PROGRAM FastTask
VAR
	_iBuffer: UDINT := 0;
END_VAR

FOR _iBuffer := 0 TO MAX_CSV_RING_BUFFER BY 1 DO
	IF gCSV_Buffer[_iBuffer].bFull THEN
		gCSV_Buffer[_iBuffer].fbWriter(bWrite:= gCSV_Buffer[_iBuffer].bFull,sFileName:=gCSV_Buffer[_iBuffer].sPath, pBuffer :=ADR(gCSV_Buffer[_iBuffer].aBuffer));
		gCSV_Buffer[_iBuffer].bFull := gCSV_Buffer[_iBuffer].fbWriter.bBusy;
	END_IF
END_FOR

END_PROGRAM
